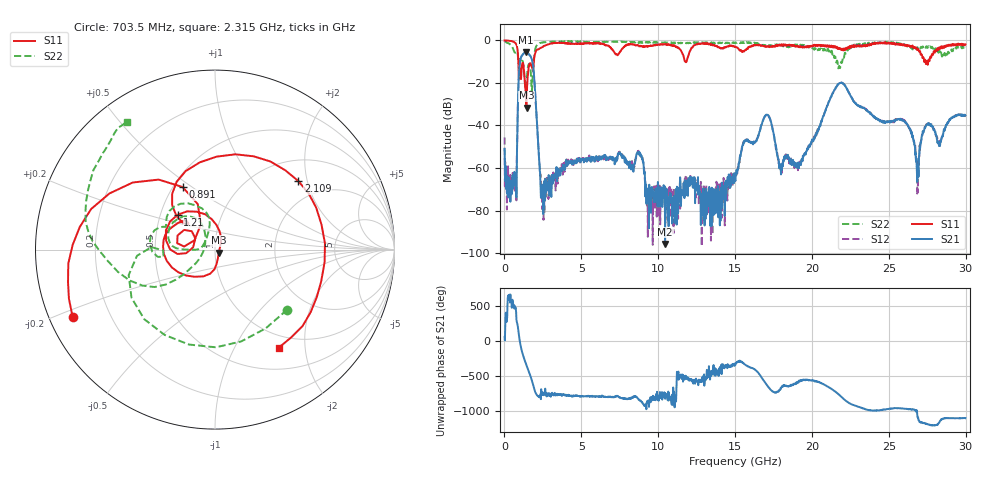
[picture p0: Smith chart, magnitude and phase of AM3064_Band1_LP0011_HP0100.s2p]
# Hz S DB R 50.0
!freq dBS11 angS11 dBS21 angS21 dBS12 angS12 dBS22 angS22
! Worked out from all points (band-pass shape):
!   1600 points, 10 MHz to 29.98 GHz, reference 50 ohm
!   highest |S21| = -5.48 dB at 1.397 GHz (marker M1); lowest = -95.7 dB at 10.45 GHz (marker M2)
!   |S21| within 3 dB of the highest: 1.058 GHz to 1.761 GHz (703.4 MHz wide, 49.9 % of centre)
!   lowest |S11| = -31.6 dB at 1.435 GHz (marker M3), VSWR 1.05, Z = 52.1 - j1.7 ohm
!   |S11| at or under -10 dB: 902 MHz to 1.913 GHz (1.011 GHz wide, 71.9 % of centre); 11.76 GHz to 11.84 GHz (80.84 MHz wide, 0.685 % of centre); 27.3932 GHz to 27.46066 GHz (67.45 MHz wide, 0.246 % of centre)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
!   |S22| runs from -24.0 to -0.3 dB; largest |S21 - S12| = 0.0064
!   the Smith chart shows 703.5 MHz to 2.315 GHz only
!   S11 on the Smith chart (normalised r, x): 703.5 MHz: 0.07, -0.22; 891 MHz: 0.56, +0.46; 1.21 GHz: 0.61, +0.26; 2.109 GHz: 1.48, +1.77; 2.315 GHz: 0.81, -1.53
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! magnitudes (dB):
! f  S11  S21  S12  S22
! 10 MHz  -0.1  -51.0  -45.6  -0.3
! 703.5 MHz  -1.1  -64.4  -70.0  -5.6
! 891 MHz  -8.1  -25.3  -25.2  -9.0
! 1.21 GHz  -10.9  -6.5  -6.5  -10.5
! 1.397 GHz  -26.5  -5.5  -5.4  -21.7
! 1.435 GHz  -31.6  -5.6  -5.5  -19.0
! 1.828 GHz  -13.5  -10.3  -10.3  -17.7
! 2.109 GHz  -4.4  -38.0  -38.2  -2.3
! 2.315 GHz  -3.7  -61.7  -63.5  -1.3
! 5.015 GHz  -1.4  -55.6  -55.8  -0.6
! 8.782 GHz  -2.6  -52.5  -52.8  -0.8
! 10 GHz  -2.0  -75.0  -74.3  -0.9
! 10.45 GHz  -1.7  -95.7  -73.9  -0.9
! 15 GHz  -3.0  -65.5  -64.2  -1.2
! 17.03 GHz  -3.1  -35.0  -34.9  -2.6
! 17.97 GHz  -2.5  -59.1  -60.9  -2.1
! 19.99 GHz  -3.0  -47.3  -48.0  -3.4
! 21.83 GHz  -3.9  -20.1  -19.9  -13.1
! 25 GHz  -1.0  -38.1  -38.3  -1.1
! 26.89 GHz  -4.1  -58.8  -71.3  -3.6
! 27.45 GHz  -10.3  -39.8  -39.4  -2.7
! 29.98 GHz  -1.9  -35.3  -35.3  -3.2
